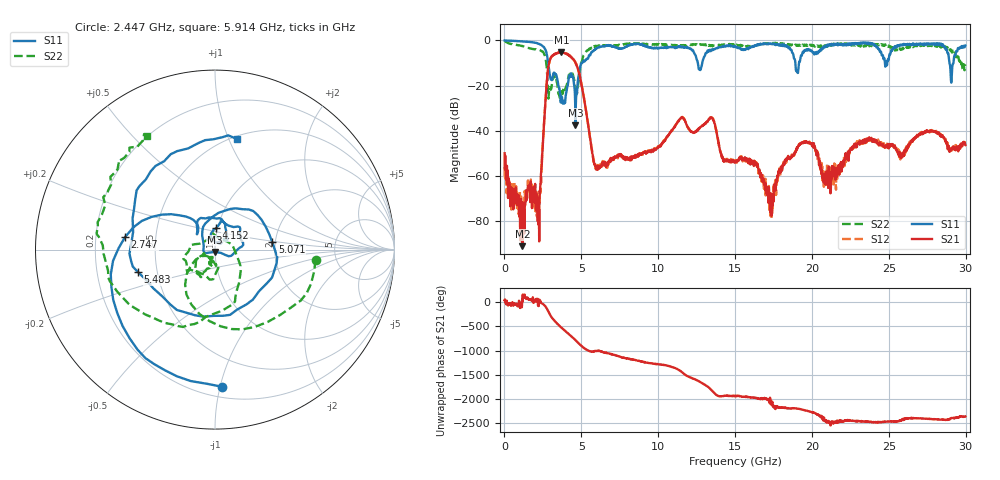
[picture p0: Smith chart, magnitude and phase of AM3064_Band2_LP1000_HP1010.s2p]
# Hz S DB R 50.0
!freq dBS11 angS11 dBS21 angS21 dBS12 angS12 dBS22 angS22
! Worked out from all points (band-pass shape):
!   1600 points, 10 MHz to 29.98 GHz, reference 50 ohm
!   highest |S21| = -5.26 dB at 3.703 GHz (marker M1); lowest = -91.2 dB at 1.172 GHz (marker M2)
!   |S21| within 3 dB of the highest: 2.98 GHz to 4.456 GHz (1.476 GHz wide, 39.7 % of centre)
!   lowest |S11| = -37.6 dB at 4.621 GHz (marker M3), VSWR 1.03, Z = 50 - j1.32 ohm
!   |S11| at or under -10 dB: 2.839 GHz to 5.058 GHz (2.218 GHz wide, 56.2 % of centre); 12.58 GHz to 12.86 GHz (284.6 MHz wide, 2.24 % of centre); 28.94 GHz to 29.2 GHz (256.6 MHz wide, 0.883 % of centre)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
!   |S22| runs from -27.2 to -0.3 dB; largest |S21 - S12| = 0.018
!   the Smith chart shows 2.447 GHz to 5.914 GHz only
!   S11 on the Smith chart (normalised r, x): 2.447 GHz: 0.28, -1.01; 2.747 GHz: 0.33, +0.06; 4.152 GHz: 0.98, +0.24; 5.071 GHz: 1.93, +0.18; 5.483 GHz: 0.39, -0.12; 5.914 GHz: 0.53, +1.07
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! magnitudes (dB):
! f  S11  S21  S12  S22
! 10 MHz  0.0  -50.1  -56.4  -0.3
! 1.172 GHz  -0.4  -91.2  -82.1  -2.5
! 2.184 GHz  -1.5  -73.7  -72.8  -4.1
! 2.447 GHz  -2.3  -51.1  -51.6  -5.0
! 2.747 GHz  -5.9  -19.3  -19.3  -11.8
! 3.703 GHz  -25.0  -5.3  -5.5  -22.7
! 4.152 GHz  -18.5  -6.5  -6.4  -16.7
! 4.621 GHz  -37.6  -9.9  -9.8  -23.2
! 5.015 GHz  -10.2  -19.5  -19.5  -9.6
! 5.071 GHz  -9.8  -21.6  -21.5  -8.5
! 5.483 GHz  -7.0  -39.2  -39.2  -4.1
! 5.914 GHz  -4.0  -55.7  -55.3  -2.6
! 10 GHz  -3.4  -47.1  -47.1  -1.8
! 13.43 GHz  -4.4  -34.2  -34.1  -2.3
! 15 GHz  -2.6  -54.3  -53.5  -1.9
! 16.35 GHz  -2.2  -54.3  -54.7  -2.3
! 17.31 GHz  -1.6  -72.2  -77.8  -1.3
! 18.29 GHz  -2.5  -53.7  -53.0  -2.0
! 19.99 GHz  -4.6  -46.2  -46.1  -1.9
! 21.12 GHz  -1.9  -59.7  -56.6  -2.5
! 25 GHz  -8.3  -47.9  -46.3  -2.3
! 29.98 GHz  -2.2  -46.4  -45.9  -10.6
